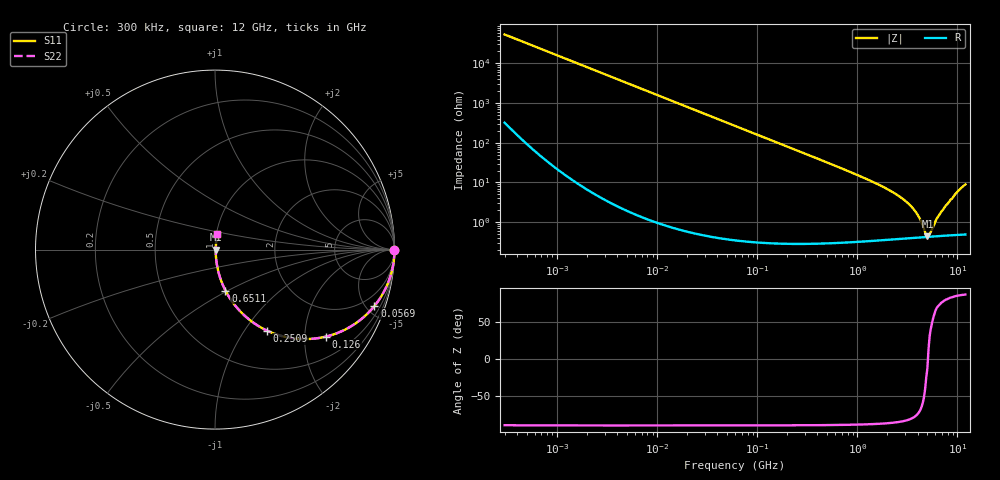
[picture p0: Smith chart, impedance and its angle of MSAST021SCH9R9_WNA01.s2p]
! MSAST021SCH9R9_WNA01  S-PARAMETER MODEL  ( General Type )
! Model Generated by TAIYO YUDEN Corporation (http://www.ty-top.com)
! Version 2.0
! TAIYO YUDEN Control No. 181101
! Copyright(c) 2015 TAIYO YUDEN CO.,LTD. All Rights Reserved.
! Product Description (link to TY-COMPAS)
! https://ds.yuden.co.jp/TYCOMPAS/or/detail?pn=MSAST021SCH9R9CWNA01&u=M
! Products Name : Multilayer Ceramic Capacitors
! Characteristics :
!  Capacitance : 9.9 pF , Rated Voltage : 25V , TCC : CH / C0H
!  Case Size : 0.25 x 0.125 / 0.0098 x 0.0049 [mm/inch] , Thickness : 0.125 / 0.0049 [mm/inch]
!  (Conditions: Temperature = 25 degC , DC Bias Current/Voltage = 0A / 0V)
! External Node Assignments :
!  1  o---| |---o  2
! GND o---------o GND
! Frequency Range : 0.3MHz  -  12000MHz  [ 401 STEP ]
# MHz S RI R 50
! Freq[MHz].  S11 Real  S11 Imag  S21 Real  S21 Imag  S12 Real  S12 Imag  S22 Real  S22 Imag
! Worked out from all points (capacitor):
!   401 points, 300 kHz to 12 GHz, reference 50 ohm
!   read as one part in series: C = 9.9 pF near 316.3 kHz
!   lowest |Z| = 437 mohm at 5.006 GHz (marker M1)
!   series resonance near 5.072 GHz, so ESL is about 99 pH
!   S11 on the Smith chart (normalised r, x): 300 kHz: open; 56.9 MHz: 1.01, -5.65; 126 MHz: 1.01, -2.55; 250.9 MHz: 1.01, -1.28; 651.1 MHz: 1.01, -0.49; 12 GHz: 1.01, +0.18
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0.3  1 -0.00187  1.47e-05 0.00187  1.47e-05 0.00187  1 -0.00187
1.769972  0.9999 -0.011  0.000131 0.011  0.000131 0.011  0.9999 -0.011
10.44266  0.9958 -0.0647  0.00424 0.0647  0.00424 0.0647  0.9958 -0.0647
25.70316  0.975 -0.1559  0.025 0.1559  0.025 0.1559  0.975 -0.1559
56.90376  0.8883 -0.3143  0.1117 0.3143  0.1117 0.3143  0.8883 -0.3143
60  0.8774 -0.3273  0.1226 0.3273  0.1226 0.3273  0.8774 -0.3273
125.9782  0.619 -0.4845  0.381 0.4845  0.381 0.4845  0.619 -0.4845
177.7716  0.4494 -0.4959  0.5506 0.4959  0.5506 0.4959  0.4494 -0.4959
250.8588  0.2909 -0.452  0.7091 0.452  0.7091 0.452  0.2909 -0.452
353.9943  0.1711 -0.3735  0.8289 0.3735  0.8289 0.3735  0.1711 -0.3735
651.0506  0.0582 -0.228  0.9418 0.228  0.9418 0.228  0.0582 -0.228
2088.533  0.0076 -0.063  0.9924 0.063  0.9924 0.063  0.0076 -0.063
2870.14  0.00523 -0.0374  0.9948 0.0374  0.9948 0.0374  0.00523 -0.0374
3547.679  0.00449 -0.0226  0.9955 0.0226  0.9955 0.0226  0.00449 -0.0226
4050.141  0.00427 -0.0139  0.9957 0.0139  0.9957 0.0139  0.00427 -0.0139
4747.894  0.00422 -0.00368  0.9958 0.00368  0.9958 0.00368  0.00422 -0.00368
5006.236  0.00424 -0.000973  0.9958 0.000973  0.9958 0.000973  0.00424 -0.000973
5278.635  0.00429 0.00258  0.9957 -0.00258  0.9957 -0.00258  0.00429 0.00258
6354.153  0.00458 0.0126  0.9954 -0.0126  0.9954 -0.0126  0.00458 0.0126
7254.098  0.00496 0.0208  0.995 -0.0208  0.995 -0.0208  0.00496 0.0208
9968.853  0.00799 0.0568  0.992 -0.0568  0.992 -0.0568  0.00799 0.0568
12000  0.0126 0.0876  0.9874 -0.0876  0.9874 -0.0876  0.0126 0.0876
